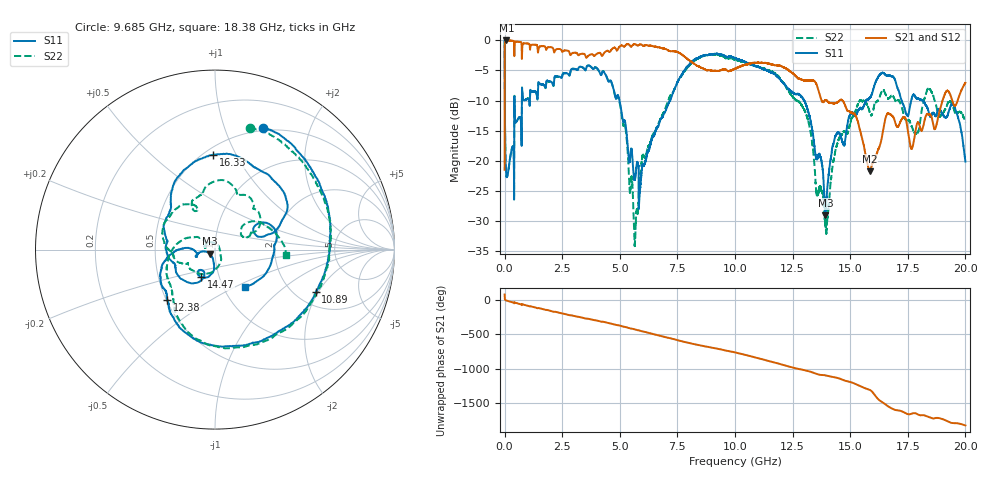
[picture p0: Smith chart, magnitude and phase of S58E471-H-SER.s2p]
!{S58E471}
!Johanson Technology Inc.
!www.johansontechnology.com
!Test Board Conditions:
!Substrate Type  RO4350B
!Substrate Thickness  60 mil
!Substrate Dk  3.66
!TL Type: GCPW
!TL Trace Width  115 mil
!TL Gap  52 mil
!Electrode orientation  Horizontal
!DUT TOPOLOGY	SERIES
!Mounting Pad LxW  55x428 mil
! Created Wed Apr 14 11:52:15 2021
# mhz S ma R 50
! 2 Port Network Data from SP1.SP block
! freq  magS11  angS11  magS21  angS21  magS12  angS12  magS22  angS22
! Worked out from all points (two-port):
!   20001 points, 300 kHz to 20 GHz, reference 50 ohm
!   highest |S21| = -0.03 dB at 81.3 MHz (marker M1); lowest = -21.7 dB at 15.84 GHz (marker M2)
!   |S21| within 3 dB of the highest: 3.587 MHz to 749.7 MHz (746.1 MHz wide, 198 % of centre); 751.9 MHz to 7.909 GHz (7.157 GHz wide, 165 % of centre)
!   lowest |S11| = -29.0 dB at 13.92 GHz (marker M3), VSWR 1.07, Z = 47.3 - j2.16 ohm
!   |S11| at or under -10 dB: 4.987 GHz to 7.182 GHz (2.195 GHz wide, 36.1 % of centre); 13.01 GHz to 15.68 GHz (2.678 GHz wide, 18.7 % of centre); 18.15 GHz to end of sweep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
!   |S22| runs from -34.1 to -0.1 dB; largest |S21 - S12| = 0.016
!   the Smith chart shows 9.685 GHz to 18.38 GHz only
!   S11 on the Smith chart (normalised r, x): 9.685 GHz: 0.48, +1.36; 10.89 GHz: 2.53, -1.91; 12.38 GHz: 0.51, -0.33; 14.47 GHz: 0.82, -0.26; 16.33 GHz: 0.56, +0.81; 18.38 GHz: 1.26, -0.56
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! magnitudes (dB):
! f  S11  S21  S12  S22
! 300 kHz  0.0  -21.5  -21.4  -0.1
! 81.3 MHz  -22.6  0.0  0.0  -22.5
! 848.3 MHz  -10.0  -0.5  -0.5  -9.9
! 3.334 GHz  -4.4  -2.2  -2.2  -4.4
! 4.962 GHz  -9.6  -1.2  -1.2  -9.7
! 5.688 GHz  -22.3  -0.7  -0.7  -31.1
! 5.976 GHz  -20.9  -0.8  -0.8  -19.2
! 6.667 GHz  -14.3  -1.2  -1.2  -13.9
! 9.685 GHz  -2.8  -5.1  -5.2  -3.0
! 10 GHz  -3.0  -4.7  -4.7  -3.2
! 10.89 GHz  -4.3  -3.8  -3.8  -4.3
! 12.38 GHz  -8.2  -5.1  -5.0  -8.7
! 13.33 GHz  -14.4  -6.7  -6.7  -16.7
! 13.92 GHz  -29.0  -9.9  -9.8  -30.5
! 14.47 GHz  -15.3  -10.2  -10.1  -16.7
! 15.84 GHz  -9.6  -21.7  -21.6  -11.9
! 16.33 GHz  -5.6  -16.9  -17.0  -8.9
! 16.67 GHz  -5.9  -12.1  -12.2  -9.6
! 17.86 GHz  -9.6  -14.6  -14.6  -15.4
! 18.38 GHz  -11.5  -12.3  -12.2  -8.0
! 19.48 GHz  -10.8  -10.6  -10.6  -11.2
! 20 GHz  -20.1  -7.1  -7.0  -13.7
